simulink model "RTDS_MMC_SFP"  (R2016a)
settings: Solver=FixedStepAuto  StartTime=0.0  StopTime=0.4  RelTol=1e-3
PreLoadFcn:
  | % --- DO NOT REMOVE THIS CODE (2024.3.b1) ---
  |     % create Simulink variants
  |     if not(exist('variant_simulation', 'var'))
  |         variant_simulation = Simulink.Variant('SIMULINK_MODE==0');
  |     end
  |     if not(exist('variant_generation', 'var'))
  |         variant_generation = Simulink.Variant('SIMULINK_MODE==1');
  |     end
  | 
  |     % check SDK version
  |     required_lib_version = 3900.3;
  |     required_lib_ver_str = '2024.3';
  |     lib_path = [getenv('IX_SIMULINK_ACG_BB_3') '\simulink\blocks\BoomBox.slx'];
  |     if exist(lib_path, 'file')
  |         lib_version = str2double(Simulink.MDLInfo(lib_path).ModelVersion); % fullpath to avoid getting shadowing files
  |         if lib_version < required_lib_version || isnan(lib_version)
  |             error(['The model ''' bdroot ''' has been saved with a more recent version of ACG SDK (' required_lib_ver_str ') and might not work as expected. <a href="matlab:private_end_string = ''--- PLACE YOUR CODE BELOW THIS LINE ---'';private_fcn = get_param(bdroot, ''PreLoadFcn'');private_end_index = strfind(private_fcn, private_end_string);set_param(bdroot, ''PreLoadFcn'', strtrim(private_fcn(private_end_index(end)+length(private_end_string):end)));private_fcn = get_param(bdroot, ''PostLoadFcn'');private_end_index = strfind(private_fcn, private_end_string);set_param(bdroot, ''PostLoadFcn'', strtrim(private_fcn(private_end_index(end)+length(private_end_string):end)));private_fcn = get_param(bdroot, ''InitFcn'');private_end_index = strfind(private_fcn, private_end_string);set_param(bdroot, ''InitFcn'', strtrim(private_fcn(private_end_index(end)+length(private_end_string):end)));clear private_end_string private_fcn private_end_index;open(bdroot);">Click here</a> to continue anyway, or download the latest version of the SDK at <a href="www.imperix.com/downloads">www.imperix.ch/downloads</a>.']);
  |         end
  |     elseif exist(getenv('IX_SIMULINK_ACG_BB_3'), 'dir')
  |         error(['Library file for imperix ACG SDK not found in path ''' lib_path '''. Please try to re-install ACG SDK (<a href="www.imperix.com/downloads">www.imperix.ch/downloads</a>).']);
  |     else
  |         error('ACG SDK is not installed on this computer and the model will not work as expected. Please download ACG SDK at <a href="www.imperix.com/downloads">www.imperix.ch/downloads</a>, install it, and reopen the model.');
  |     end
  |     clear required_lib_version required_lib_ver_str lib_path lib_version;
  | 
  |     ix_acg_path = getenv('IX_SIMULINK_ACG_BB_3');
  |     addpath(fullfile(ix_acg_path, 'simulink\target'));
  |     addpath(fullfile(ix_acg_path, 'simulink\blocks'));
  |     addpath(fullfile(ix_acg_path, 'simulink\functions'));
  |     sl_refresh_customizations;
  |     clear ix_acg_path;
  | 
  |     % The SIMULINK_MODE variable is created in the base
  |     % workspace in the PostLoadFcn from the block whose id is kb0101
  |     % All opened models share a common variant configuration.
  | 
  |     Model_PreLoadFcn(bdroot);
  | % --- PLACE YOUR CODE BELOW THIS LINE ---
PostLoadFcn:
  | % --- DO NOT REMOVE THIS CODE (2024.3.b1) ---
  |     % change the execution mode of simulink depending on the radio button:
  |     if(strcmp('Automated Code Generation',get_param(Find_imperix_blocks(bdroot,'Configuration'),'SLMODE')))
  |         assignin('base', 'SIMULINK_MODE', 1);
  |     else
  |         assignin('base', 'SIMULINK_MODE', 0);
  |     end
  | 
  |     Model_PostLoadFcn(bdroot);
  | % --- PLACE YOUR CODE BELOW THIS LINE ---
InitFcn:
  | % --- DO NOT REMOVE THIS CODE (2024.3.b1) ---
  |     % check SDK version
  |     required_lib_version = 3900.3;
  |     required_lib_ver_str = '2024.3';
  |     lib_path = [getenv('IX_SIMULINK_ACG_BB_3') '\simulink\blocks\BoomBox.slx'];
  |     if exist(lib_path, 'file')
  |         lib_version = str2double(Simulink.MDLInfo(lib_path).ModelVersion); % fullpath to avoid getting shadowing files
  |         if lib_version < required_lib_version || isnan(lib_version)
  |             error(['The model ''' bdroot ''' has been saved with a more recent version of ACG SDK (' required_lib_ver_str ') and might not work as expected. <a href="matlab:private_end_string = ''--- PLACE YOUR CODE BELOW THIS LINE ---'';private_fcn = get_param(bdroot, ''PreLoadFcn'');private_end_index = strfind(private_fcn, private_end_string);set_param(bdroot, ''PreLoadFcn'', strtrim(private_fcn(private_end_index(end)+length(private_end_string):end)));private_fcn = get_param(bdroot, ''PostLoadFcn'');private_end_index = strfind(private_fcn, private_end_string);set_param(bdroot, ''PostLoadFcn'', strtrim(private_fcn(private_end_index(end)+length(private_end_string):end)));private_fcn = get_param(bdroot, ''InitFcn'');private_end_index = strfind(private_fcn, private_end_string);set_param(bdroot, ''InitFcn'', strtrim(private_fcn(private_end_index(end)+length(private_end_string):end)));clear private_end_string private_fcn private_end_index;open(bdroot);">Click here</a> to continue anyway, or download the latest version of the SDK at <a href="www.imperix.com/downloads">www.imperix.ch/downloads</a>.']);
  |         end
  |     elseif exist(getenv('IX_SIMULINK_ACG_BB_3'), 'dir')
  |         error(['Library file for imperix ACG SDK not found in path ''' lib_path '''. Please try to re-install ACG SDK (<a href="www.imperix.com/downloads">www.imperix.ch/downloads</a>).']);
  |     else
  |         error('ACG SDK is not installed on this computer and the model will not work as expected. Please download ACG SDK at <a href="www.imperix.com/downloads">www.imperix.ch/downloads</a>, install it, and reopen the model.');
  |     end
  |     clear required_lib_version required_lib_ver_str lib_path lib_version;
  | 
  |     Model_InitFcn(bdroot);
  | % --- PLACE YOUR CODE BELOW THIS LINE ---
model workspace (MAT data in the model file):
  CTRLPERIOD = 0.0002
  TSAMPLE = 2e-06
  global_CLK_number = 0
  global_INT_number = 1
  global_SVM_instance_id = 0
  global_can_baud_rate = '1000000'
  global_comp_time = 0.2
  global_cycle_delay = 8e-05
  global_ip_addresses : cell (value not decoded)
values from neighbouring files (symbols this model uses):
  Ki_Vleg = 1/Ti    (= 2.95256991686)    [RTDS_MMC_SFP_init.m]
  Kp_Vleg = Tn/Ti    (= 0.14880952381)    [RTDS_MMC_SFP_init.m]
  N = 4    [RTDS_MMC_SFP_init.m]
  scale_factor = 0.5^16    (= 1.52587890625e-05)    [RTDS_MMC_SFP_init.m]
  Tsw = 1/fsw    (= 0.0008)    [RTDS_MMC_SFP_init.m]
  Vsm_max = 250    [RTDS_MMC_SFP_init.m]
undefined symbols (not defined in the file or in its folder): B, Board, Box, channel, DT, lane, Micro, ns, PRO, RCP, TPI, Vf
libraries: BoomBox x183, simulink x55
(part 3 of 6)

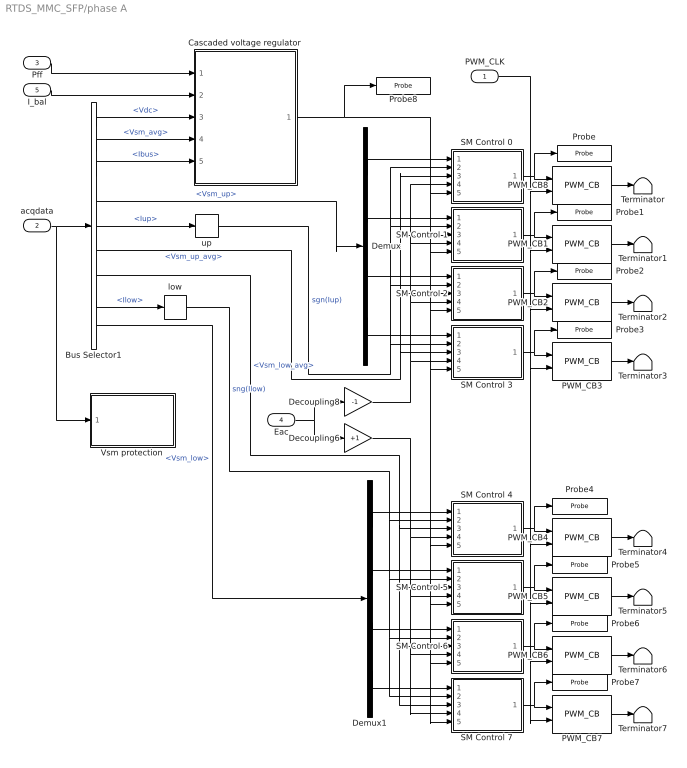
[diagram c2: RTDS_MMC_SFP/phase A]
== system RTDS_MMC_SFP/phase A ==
  PWM_CLK : Inport
  acqdata : Inport  Port=2
  Pff : Inport  Port=3
  Eac : Inport  Port=4
  I_bal : Inport  Port=5
  Bus Selector1 : BusSelector  OutputSignals=Vdc,A.Vsm.Vsm_avg,A.Ibus,A.Vsm.Vsm_up,A.Iup,A.Vsm.Vsm_up_avg,A.Vsm.Vsm_low_avg,A.Ilow,A.Vsm.Vsm_low
  Cascaded voltage regulator : Subsystem
  Decoupling6 : Gain  Gain=+1
  Decoupling8 : Gain  Gain=-1
  Demux : Demux
  Demux1 : Demux
  PWM_CB1 : BoomBox/PWM_CB  NB_BBX=0  OUTCONF=Single  PWM_OUT_SINGLE=lane 1 (channel 0L)  PWM_OUT_DUAL=channel 0 (lanes 0 & 1)  CARRIER=TRIANGLE  DUTY=0  DUTY_is_RT=on  PHASE=0.25  PHASE_is_RT=off  ENABLE_is_RT=off  RATE=Double-rate  ENABLE_DOUT=PWM signals  DEADTIME=400e-9  DEADTIME_SIM=off  LNorCH_NBR=1  CH_NBR=0  LN_NBR=1  Parameter16=0  KBID=kb0401
  PWM_CB2 : BoomBox/PWM_CB  NB_BBX=0  OUTCONF=Single  PWM_OUT_SINGLE=lane 2 (channel 1H)  PWM_OUT_DUAL=channel 0 (lanes 0 & 1)  CARRIER=TRIANGLE  DUTY=0  DUTY_is_RT=on  PHASE=0.5  PHASE_is_RT=off  ENABLE_is_RT=off  RATE=Double-rate  ENABLE_DOUT=PWM signals  DEADTIME=400e-9  DEADTIME_SIM=off  LNorCH_NBR=2  CH_NBR=0  LN_NBR=2  Parameter16=0  KBID=kb0401
  PWM_CB3 : BoomBox/PWM_CB  NB_BBX=0  OUTCONF=Single  PWM_OUT_SINGLE=lane 3 (channel 1L)  PWM_OUT_DUAL=channel 0 (lanes 0 & 1)  CARRIER=TRIANGLE  DUTY=0  DUTY_is_RT=on  PHASE=0.75  PHASE_is_RT=off  ENABLE_is_RT=off  RATE=Double-rate  ENABLE_DOUT=PWM signals  DEADTIME=400e-9  DEADTIME_SIM=off  LNorCH_NBR=3  CH_NBR=0  LN_NBR=3  Parameter16=0  KBID=kb0401
  PWM_CB4 : BoomBox/PWM_CB  NB_BBX=0  OUTCONF=Single  PWM_OUT_SINGLE=lane 4 (channel 2H)  PWM_OUT_DUAL=channel 0 (lanes 0 & 1)  CARRIER=TRIANGLE  DUTY=0  DUTY_is_RT=on  PHASE=0  PHASE_is_RT=off  ENABLE_is_RT=off  RATE=Double-rate  ENABLE_DOUT=PWM signals  DEADTIME=400e-9  DEADTIME_SIM=off  LNorCH_NBR=4  CH_NBR=0  LN_NBR=4  Parameter16=0  KBID=kb0401
  PWM_CB5 : BoomBox/PWM_CB  NB_BBX=0  OUTCONF=Single  PWM_OUT_SINGLE=lane 5 (channel 2L)  PWM_OUT_DUAL=channel 0 (lanes 0 & 1)  CARRIER=TRIANGLE  DUTY=0  DUTY_is_RT=on  PHASE=0.25  PHASE_is_RT=off  ENABLE_is_RT=off  RATE=Double-rate  ENABLE_DOUT=PWM signals  DEADTIME=400e-9  DEADTIME_SIM=off  LNorCH_NBR=5  CH_NBR=0  LN_NBR=5  Parameter16=0  KBID=kb0401
  PWM_CB6 : BoomBox/PWM_CB  NB_BBX=0  OUTCONF=Single  PWM_OUT_SINGLE=lane 6 (channel 3H)  PWM_OUT_DUAL=channel 0 (lanes 0 & 1)  CARRIER=TRIANGLE  DUTY=0  DUTY_is_RT=on  PHASE=0.5  PHASE_is_RT=off  ENABLE_is_RT=off  RATE=Double-rate  ENABLE_DOUT=PWM signals  DEADTIME=400e-9  DEADTIME_SIM=off  LNorCH_NBR=6  CH_NBR=0  LN_NBR=6  Parameter16=0  KBID=kb0401
  PWM_CB7 : BoomBox/PWM_CB  NB_BBX=0  OUTCONF=Single  PWM_OUT_SINGLE=lane 7 (channel 3L)  PWM_OUT_DUAL=channel 0 (lanes 0 & 1)  CARRIER=TRIANGLE  DUTY=0  DUTY_is_RT=on  PHASE=0.75  PHASE_is_RT=off  ENABLE_is_RT=off  RATE=Double-rate  ENABLE_DOUT=PWM signals  DEADTIME=400e-9  DEADTIME_SIM=off  LNorCH_NBR=7  CH_NBR=0  LN_NBR=7  Parameter16=0  KBID=kb0401
  PWM_CB8 : BoomBox/PWM_CB  NB_BBX=0  OUTCONF=Single  PWM_OUT_SINGLE=lane 0 (channel 0H)  PWM_OUT_DUAL=channel 0 (lanes 0 & 1)  CARRIER=TRIANGLE  DUTY=0  DUTY_is_RT=on  PHASE=0  PHASE_is_RT=off  ENABLE_is_RT=off  RATE=Double-rate  ENABLE_DOUT=PWM signals  DEADTIME=400e-9  DEADTIME_SIM=off  LNorCH_NBR=0  CH_NBR=0  LN_NBR=0  Parameter16=0  KBID=kb0401
  Probe : BoomBox/Probe  VARNAME=m_A0  EVALUATE=Literal  DATATYPE=single  CAN_ENABLED=off  CAN_ADDRESS=0  CAN_TX_FREQ=10  init_baudrate=0  CAN_BAUDRATE=1000000  can_endianness=Little-endian  ETH_ENABLED=off  ETH_PORT=2000  ETH_IP_LIST=IP address 0  eth_endianness=Little-endian  ETH_TX_FREQ=10  init_ip=0  KBID=kb0502  CAN_BIG_ENDIAN=0  ETH_BIG_ENDIAN=0  ETH_IP_SFCN=empty  CAN_MB_ID=0  ETH_MB_ID=1  RESIZE=0
  Probe1 : BoomBox/Probe  VARNAME=m_A1  EVALUATE=Literal  DATATYPE=single  CAN_ENABLED=off  CAN_ADDRESS=0  CAN_TX_FREQ=10  init_baudrate=0  CAN_BAUDRATE=1000000  can_endianness=Little-endian  ETH_ENABLED=off  ETH_PORT=2000  ETH_IP_LIST=IP address 0  eth_endianness=Little-endian  ETH_TX_FREQ=10  init_ip=0  KBID=kb0502  CAN_BIG_ENDIAN=0  ETH_BIG_ENDIAN=0  ETH_IP_SFCN=empty  CAN_MB_ID=0  ETH_MB_ID=1  RESIZE=0
  Probe2 : BoomBox/Probe  VARNAME=m_A2  EVALUATE=Literal  DATATYPE=single  CAN_ENABLED=off  CAN_ADDRESS=0  CAN_TX_FREQ=10  init_baudrate=0  CAN_BAUDRATE=1000000  can_endianness=Little-endian  ETH_ENABLED=off  ETH_PORT=2000  ETH_IP_LIST=IP address 0  eth_endianness=Little-endian  ETH_TX_FREQ=10  init_ip=0  KBID=kb0502  CAN_BIG_ENDIAN=0  ETH_BIG_ENDIAN=0  ETH_IP_SFCN=empty  CAN_MB_ID=0  ETH_MB_ID=1  RESIZE=0
  Probe3 : BoomBox/Probe  VARNAME=m_A3  EVALUATE=Literal  DATATYPE=single  CAN_ENABLED=off  CAN_ADDRESS=0  CAN_TX_FREQ=10  init_baudrate=0  CAN_BAUDRATE=1000000  can_endianness=Little-endian  ETH_ENABLED=off  ETH_PORT=2000  ETH_IP_LIST=IP address 0  eth_endianness=Little-endian  ETH_TX_FREQ=10  init_ip=0  KBID=kb0502  CAN_BIG_ENDIAN=0  ETH_BIG_ENDIAN=0  ETH_IP_SFCN=empty  CAN_MB_ID=0  ETH_MB_ID=1  RESIZE=0
  Probe4 : BoomBox/Probe  VARNAME=m_A4  EVALUATE=Literal  DATATYPE=single  CAN_ENABLED=off  CAN_ADDRESS=0  CAN_TX_FREQ=10  init_baudrate=0  CAN_BAUDRATE=1000000  can_endianness=Little-endian  ETH_ENABLED=off  ETH_PORT=2000  ETH_IP_LIST=IP address 0  eth_endianness=Little-endian  ETH_TX_FREQ=10  init_ip=0  KBID=kb0502  CAN_BIG_ENDIAN=0  ETH_BIG_ENDIAN=0  ETH_IP_SFCN=empty  CAN_MB_ID=0  ETH_MB_ID=1  RESIZE=0
  Probe5 : BoomBox/Probe  VARNAME=m_A5  EVALUATE=Literal  DATATYPE=single  CAN_ENABLED=off  CAN_ADDRESS=0  CAN_TX_FREQ=10  init_baudrate=0  CAN_BAUDRATE=1000000  can_endianness=Little-endian  ETH_ENABLED=off  ETH_PORT=2000  ETH_IP_LIST=IP address 0  eth_endianness=Little-endian  ETH_TX_FREQ=10  init_ip=0  KBID=kb0502  CAN_BIG_ENDIAN=0  ETH_BIG_ENDIAN=0  ETH_IP_SFCN=empty  CAN_MB_ID=0  ETH_MB_ID=1  RESIZE=0
  Probe6 : BoomBox/Probe  VARNAME=m_A6  EVALUATE=Literal  DATATYPE=single  CAN_ENABLED=off  CAN_ADDRESS=0  CAN_TX_FREQ=10  init_baudrate=0  CAN_BAUDRATE=1000000  can_endianness=Little-endian  ETH_ENABLED=off  ETH_PORT=2000  ETH_IP_LIST=IP address 0  eth_endianness=Little-endian  ETH_TX_FREQ=10  init_ip=0  KBID=kb0502  CAN_BIG_ENDIAN=0  ETH_BIG_ENDIAN=0  ETH_IP_SFCN=empty  CAN_MB_ID=0  ETH_MB_ID=1  RESIZE=0
  Probe7 : BoomBox/Probe  VARNAME=m_A7  EVALUATE=Literal  DATATYPE=single  CAN_ENABLED=off  CAN_ADDRESS=0  CAN_TX_FREQ=10  init_baudrate=0  CAN_BAUDRATE=1000000  can_endianness=Little-endian  ETH_ENABLED=off  ETH_PORT=2000  ETH_IP_LIST=IP address 0  eth_endianness=Little-endian  ETH_TX_FREQ=10  init_ip=0  KBID=kb0502  CAN_BIG_ENDIAN=0  ETH_BIG_ENDIAN=0  ETH_IP_SFCN=empty  CAN_MB_ID=0  ETH_MB_ID=1  RESIZE=0
  Probe8 : BoomBox/Probe  VARNAME=Edc_A  EVALUATE=Literal  DATATYPE=single  CAN_ENABLED=off  CAN_ADDRESS=0  CAN_TX_FREQ=10  init_baudrate=0  CAN_BAUDRATE=1000000  can_endianness=Little-endian  ETH_ENABLED=off  ETH_PORT=2000  ETH_IP_LIST=IP address 0  eth_endianness=Little-endian  ETH_TX_FREQ=10  init_ip=0  KBID=kb0502  CAN_BIG_ENDIAN=0  ETH_BIG_ENDIAN=0  ETH_IP_SFCN=empty  CAN_MB_ID=0  ETH_MB_ID=1  RESIZE=0
  SM Control 0 : Subsystem
  SM Control 1 : Subsystem
  SM Control 2 : Subsystem
  SM Control 3 : Subsystem
  SM Control 4 : Subsystem
  SM Control 5 : Subsystem
  SM Control 6 : Subsystem
  SM Control 7 : Subsystem
  Terminator{,1..7} (8 alike) : Terminator
  Vsm protection : Subsystem
  low : Signum
  up : Signum
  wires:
  low/1 -> SM Control 4/2(sign), SM Control 5/2(sign), SM Control 7/2(sign), SM Control 6/2(sign)  "sng(Ilow)"
  Bus Selector1/6 -> SM Control 3/3(Vsm_avg), SM Control 2/3(Vsm_avg), SM Control 1/3(Vsm_avg), SM Control 0/3(Vsm_avg)  "<Vsm_up_avg>"
  Demux1/1 -> SM Control 4/1(Vsm)
  Demux/3 -> SM Control 2/1(Vsm)
  Demux/2 -> SM Control 1/1(Vsm)
  Demux/4 -> SM Control 3/1(Vsm)
  Decoupling8/1 -> SM Control 3/4(Eac), SM Control 2/4(Eac), SM Control 1/4(Eac), SM Control 0/4(Eac)
  up/1 -> SM Control 3/2(sign), SM Control 2/2(sign), SM Control 1/2(sign), SM Control 0/2(sign)  "sgn(Iup)"
  acqdata/1 -> Vsm protection/1(acqdata), Bus Selector1/1
  Demux1/2 -> SM Control 5/1(Vsm)
  PWM_CLK/1 -> PWM_CB8/2, PWM_CB1/2, PWM_CB2/2, PWM_CB3/2, PWM_CB4/2, PWM_CB5/2, PWM_CB7/2, PWM_CB6/2
  SM Control 1/1(m) -> PWM_CB1/1, Probe1/1
  Demux1/4 -> SM Control 7/1(Vsm)
  SM Control 6/1(m) -> PWM_CB6/1, Probe6/1
  Decoupling6/1 -> SM Control 4/4(Eac), SM Control 5/4(Eac), SM Control 7/4(Eac), SM Control 6/4(Eac)
  Bus Selector1/7 -> SM Control 4/3(Vsm_avg), SM Control 5/3(Vsm_avg), SM Control 7/3(Vsm_avg), SM Control 6/3(Vsm_avg)  "<Vsm_low_avg>"
  Bus Selector1/8 -> low/1  "<Ilow>"
  Bus Selector1/9 -> Demux1/1  "<Vsm_low>"
  Demux/1 -> SM Control 0/1(Vsm)
  SM Control 5/1(m) -> PWM_CB5/1, Probe5/1
  SM Control 7/1(m) -> PWM_CB7/1, Probe7/1
  SM Control 3/1(m) -> PWM_CB3/1, Probe3/1
  Demux1/3 -> SM Control 6/1(Vsm)
  SM Control 0/1(m) -> Probe/1, PWM_CB8/1
  SM Control 2/1(m) -> PWM_CB2/1, Probe2/1
  SM Control 4/1(m) -> PWM_CB4/1, Probe4/1
  Bus Selector1/4 -> Demux/1  "<Vsm_up>"
  Bus Selector1/5 -> up/1  "<Iup>"
  Eac/1 -> Decoupling6/1, Decoupling8/1
  Cascaded voltage regulator/1(Edc) -> Probe8/1, SM Control 1/5(Edc), SM Control 2/5(Edc), SM Control 3/5(Edc), SM Control 4/5(Edc), SM Control 5/5(Edc), SM Control 7/5(Edc), SM Control 6/5(Edc), SM Control 0/5(Edc)
  Pff/1 -> Cascaded voltage regulator/1(Pff)
  I_bal/1 -> Cascaded voltage regulator/2(I_bal)
  Bus Selector1/1 -> Cascaded voltage regulator/3(Vdc)  "<Vdc>"
  Bus Selector1/2 -> Cascaded voltage regulator/4(Vsm_avg)  "<Vsm_avg>"
  Bus Selector1/3 -> Cascaded voltage regulator/5(Ibus)  "<Ibus>"
  PWM_CB8/1 -> Terminator/1
  PWM_CB1/1 -> Terminator1/1
  PWM_CB3/1 -> Terminator3/1
  PWM_CB2/1 -> Terminator2/1
  PWM_CB5/1 -> Terminator5/1
  PWM_CB4/1 -> Terminator4/1
  PWM_CB6/1 -> Terminator6/1
  PWM_CB7/1 -> Terminator7/1

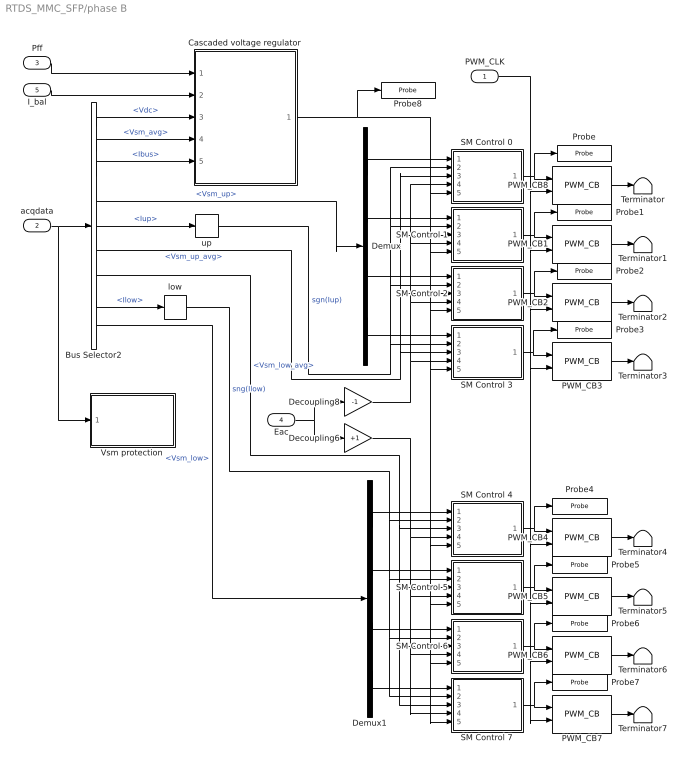
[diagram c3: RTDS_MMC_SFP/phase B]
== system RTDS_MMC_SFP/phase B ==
  PWM_CLK : Inport
  acqdata : Inport  Port=2
  Pff : Inport  Port=3
  Eac : Inport  Port=4
  I_bal : Inport  Port=5
  Bus Selector2 : BusSelector  OutputSignals=Vdc,B.Vsm.Vsm_avg,B.Ibus,B.Vsm.Vsm_up,B.Iup,B.Vsm.Vsm_up_avg,B.Vsm.Vsm_low_avg,B.Ilow,B.Vsm.Vsm_low
  Cascaded voltage regulator : Subsystem
  Decoupling6 : Gain  Gain=+1
  Decoupling8 : Gain  Gain=-1
  Demux : Demux
  Demux1 : Demux
  PWM_CB1 : BoomBox/PWM_CB  NB_BBX=0  OUTCONF=Single  PWM_OUT_SINGLE=lane 9 (channel 4L)  PWM_OUT_DUAL=channel 0 (lanes 0 & 1)  CARRIER=TRIANGLE  DUTY=0  DUTY_is_RT=on  PHASE=0.25  PHASE_is_RT=off  ENABLE_is_RT=off  RATE=Double-rate  ENABLE_DOUT=PWM signals  DEADTIME=400e-9  DEADTIME_SIM=off  LNorCH_NBR=9  CH_NBR=0  LN_NBR=9  Parameter16=0  KBID=kb0401
  PWM_CB2 : BoomBox/PWM_CB  NB_BBX=0  OUTCONF=Single  PWM_OUT_SINGLE=lane 10 (channel 5H)  PWM_OUT_DUAL=channel 0 (lanes 0 & 1)  CARRIER=TRIANGLE  DUTY=0  DUTY_is_RT=on  PHASE=0.5  PHASE_is_RT=off  ENABLE_is_RT=off  RATE=Double-rate  ENABLE_DOUT=PWM signals  DEADTIME=400e-9  DEADTIME_SIM=off  LNorCH_NBR=10  CH_NBR=0  LN_NBR=10  Parameter16=0  KBID=kb0401
  PWM_CB3 : BoomBox/PWM_CB  NB_BBX=0  OUTCONF=Single  PWM_OUT_SINGLE=lane 11 (channel 5L)  PWM_OUT_DUAL=channel 0 (lanes 0 & 1)  CARRIER=TRIANGLE  DUTY=0  DUTY_is_RT=on  PHASE=0.75  PHASE_is_RT=off  ENABLE_is_RT=off  RATE=Double-rate  ENABLE_DOUT=PWM signals  DEADTIME=400e-9  DEADTIME_SIM=off  LNorCH_NBR=11  CH_NBR=0  LN_NBR=11  Parameter16=0  KBID=kb0401
  PWM_CB4 : BoomBox/PWM_CB  NB_BBX=0  OUTCONF=Single  PWM_OUT_SINGLE=lane 12 (channel 6H)  PWM_OUT_DUAL=channel 0 (lanes 0 & 1)  CARRIER=TRIANGLE  DUTY=0  DUTY_is_RT=on  PHASE=0  PHASE_is_RT=off  ENABLE_is_RT=off  RATE=Double-rate  ENABLE_DOUT=PWM signals  DEADTIME=400e-9  DEADTIME_SIM=off  LNorCH_NBR=12  CH_NBR=0  LN_NBR=12  Parameter16=0  KBID=kb0401
  PWM_CB5 : BoomBox/PWM_CB  NB_BBX=0  OUTCONF=Single  PWM_OUT_SINGLE=lane 13 (channel 6L)  PWM_OUT_DUAL=channel 0 (lanes 0 & 1)  CARRIER=TRIANGLE  DUTY=0  DUTY_is_RT=on  PHASE=0.25  PHASE_is_RT=off  ENABLE_is_RT=off  RATE=Double-rate  ENABLE_DOUT=PWM signals  DEADTIME=400e-9  DEADTIME_SIM=off  LNorCH_NBR=13  CH_NBR=0  LN_NBR=13  Parameter16=0  KBID=kb0401
  PWM_CB6 : BoomBox/PWM_CB  NB_BBX=0  OUTCONF=Single  PWM_OUT_SINGLE=lane 14 (channel 7H)  PWM_OUT_DUAL=channel 0 (lanes 0 & 1)  CARRIER=TRIANGLE  DUTY=0  DUTY_is_RT=on  PHASE=0.5  PHASE_is_RT=off  ENABLE_is_RT=off  RATE=Double-rate  ENABLE_DOUT=PWM signals  DEADTIME=400e-9  DEADTIME_SIM=off  LNorCH_NBR=14  CH_NBR=0  LN_NBR=14  Parameter16=0  KBID=kb0401
  PWM_CB7 : BoomBox/PWM_CB  NB_BBX=0  OUTCONF=Single  PWM_OUT_SINGLE=lane 15 (channel 7L)  PWM_OUT_DUAL=channel 0 (lanes 0 & 1)  CARRIER=TRIANGLE  DUTY=0  DUTY_is_RT=on  PHASE=0.75  PHASE_is_RT=off  ENABLE_is_RT=off  RATE=Double-rate  ENABLE_DOUT=PWM signals  DEADTIME=400e-9  DEADTIME_SIM=off  LNorCH_NBR=15  CH_NBR=0  LN_NBR=15  Parameter16=0  KBID=kb0401
  PWM_CB8 : BoomBox/PWM_CB  NB_BBX=0  OUTCONF=Single  PWM_OUT_SINGLE=lane 8 (channel 4H)  PWM_OUT_DUAL=channel 0 (lanes 0 & 1)  CARRIER=TRIANGLE  DUTY=0  DUTY_is_RT=on  PHASE=0  PHASE_is_RT=off  ENABLE_is_RT=off  RATE=Double-rate  ENABLE_DOUT=PWM signals  DEADTIME=400e-9  DEADTIME_SIM=off  LNorCH_NBR=8  CH_NBR=0  LN_NBR=8  Parameter16=0  KBID=kb0401
  Probe : BoomBox/Probe  VARNAME=m_B0  EVALUATE=Literal  DATATYPE=single  CAN_ENABLED=off  CAN_ADDRESS=0  CAN_TX_FREQ=10  init_baudrate=0  CAN_BAUDRATE=1000000  can_endianness=Little-endian  ETH_ENABLED=off  ETH_PORT=2000  ETH_IP_LIST=IP address 0  eth_endianness=Little-endian  ETH_TX_FREQ=10  init_ip=0  KBID=kb0502  CAN_BIG_ENDIAN=0  ETH_BIG_ENDIAN=0  ETH_IP_SFCN=empty  CAN_MB_ID=0  ETH_MB_ID=1  RESIZE=0
  Probe1 : BoomBox/Probe  VARNAME=m_B1  EVALUATE=Literal  DATATYPE=single  CAN_ENABLED=off  CAN_ADDRESS=0  CAN_TX_FREQ=10  init_baudrate=0  CAN_BAUDRATE=1000000  can_endianness=Little-endian  ETH_ENABLED=off  ETH_PORT=2000  ETH_IP_LIST=IP address 0  eth_endianness=Little-endian  ETH_TX_FREQ=10  init_ip=0  KBID=kb0502  CAN_BIG_ENDIAN=0  ETH_BIG_ENDIAN=0  ETH_IP_SFCN=empty  CAN_MB_ID=0  ETH_MB_ID=1  RESIZE=0
  Probe2 : BoomBox/Probe  VARNAME=m_B2  EVALUATE=Literal  DATATYPE=single  CAN_ENABLED=off  CAN_ADDRESS=0  CAN_TX_FREQ=10  init_baudrate=0  CAN_BAUDRATE=1000000  can_endianness=Little-endian  ETH_ENABLED=off  ETH_PORT=2000  ETH_IP_LIST=IP address 0  eth_endianness=Little-endian  ETH_TX_FREQ=10  init_ip=0  KBID=kb0502  CAN_BIG_ENDIAN=0  ETH_BIG_ENDIAN=0  ETH_IP_SFCN=empty  CAN_MB_ID=0  ETH_MB_ID=1  RESIZE=0
  Probe3 : BoomBox/Probe  VARNAME=m_B3  EVALUATE=Literal  DATATYPE=single  CAN_ENABLED=off  CAN_ADDRESS=0  CAN_TX_FREQ=10  init_baudrate=0  CAN_BAUDRATE=1000000  can_endianness=Little-endian  ETH_ENABLED=off  ETH_PORT=2000  ETH_IP_LIST=IP address 0  eth_endianness=Little-endian  ETH_TX_FREQ=10  init_ip=0  KBID=kb0502  CAN_BIG_ENDIAN=0  ETH_BIG_ENDIAN=0  ETH_IP_SFCN=empty  CAN_MB_ID=0  ETH_MB_ID=1  RESIZE=0
  Probe4 : BoomBox/Probe  VARNAME=m_B4  EVALUATE=Literal  DATATYPE=single  CAN_ENABLED=off  CAN_ADDRESS=0  CAN_TX_FREQ=10  init_baudrate=0  CAN_BAUDRATE=1000000  can_endianness=Little-endian  ETH_ENABLED=off  ETH_PORT=2000  ETH_IP_LIST=IP address 0  eth_endianness=Little-endian  ETH_TX_FREQ=10  init_ip=0  KBID=kb0502  CAN_BIG_ENDIAN=0  ETH_BIG_ENDIAN=0  ETH_IP_SFCN=empty  CAN_MB_ID=0  ETH_MB_ID=1  RESIZE=0
  Probe5 : BoomBox/Probe  VARNAME=m_B5  EVALUATE=Literal  DATATYPE=single  CAN_ENABLED=off  CAN_ADDRESS=0  CAN_TX_FREQ=10  init_baudrate=0  CAN_BAUDRATE=1000000  can_endianness=Little-endian  ETH_ENABLED=off  ETH_PORT=2000  ETH_IP_LIST=IP address 0  eth_endianness=Little-endian  ETH_TX_FREQ=10  init_ip=0  KBID=kb0502  CAN_BIG_ENDIAN=0  ETH_BIG_ENDIAN=0  ETH_IP_SFCN=empty  CAN_MB_ID=0  ETH_MB_ID=1  RESIZE=0
  Probe6 : BoomBox/Probe  VARNAME=m_B6  EVALUATE=Literal  DATATYPE=single  CAN_ENABLED=off  CAN_ADDRESS=0  CAN_TX_FREQ=10  init_baudrate=0  CAN_BAUDRATE=1000000  can_endianness=Little-endian  ETH_ENABLED=off  ETH_PORT=2000  ETH_IP_LIST=IP address 0  eth_endianness=Little-endian  ETH_TX_FREQ=10  init_ip=0  KBID=kb0502  CAN_BIG_ENDIAN=0  ETH_BIG_ENDIAN=0  ETH_IP_SFCN=empty  CAN_MB_ID=0  ETH_MB_ID=1  RESIZE=0
  Probe7 : BoomBox/Probe  VARNAME=m_B7  EVALUATE=Literal  DATATYPE=single  CAN_ENABLED=off  CAN_ADDRESS=0  CAN_TX_FREQ=10  init_baudrate=0  CAN_BAUDRATE=1000000  can_endianness=Little-endian  ETH_ENABLED=off  ETH_PORT=2000  ETH_IP_LIST=IP address 0  eth_endianness=Little-endian  ETH_TX_FREQ=10  init_ip=0  KBID=kb0502  CAN_BIG_ENDIAN=0  ETH_BIG_ENDIAN=0  ETH_IP_SFCN=empty  CAN_MB_ID=0  ETH_MB_ID=1  RESIZE=0
  Probe8 : BoomBox/Probe  VARNAME=Edc_B  EVALUATE=Literal  DATATYPE=single  CAN_ENABLED=off  CAN_ADDRESS=0  CAN_TX_FREQ=10  init_baudrate=0  CAN_BAUDRATE=1000000  can_endianness=Little-endian  ETH_ENABLED=off  ETH_PORT=2000  ETH_IP_LIST=IP address 0  eth_endianness=Little-endian  ETH_TX_FREQ=10  init_ip=0  KBID=kb0502  CAN_BIG_ENDIAN=0  ETH_BIG_ENDIAN=0  ETH_IP_SFCN=empty  CAN_MB_ID=0  ETH_MB_ID=1  RESIZE=0
  SM Control 0 : Subsystem
  SM Control 1 : Subsystem
  SM Control 2 : Subsystem
  SM Control 3 : Subsystem
  SM Control 4 : Subsystem
  SM Control 5 : Subsystem
  SM Control 6 : Subsystem
  SM Control 7 : Subsystem
  Terminator{,1..7} (8 alike) : Terminator
  Vsm protection : Subsystem
  low : Signum
  up : Signum
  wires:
  Bus Selector2/3 -> Cascaded voltage regulator/5(Ibus)  "<Ibus>"
  Bus Selector2/2 -> Cascaded voltage regulator/4(Vsm_avg)  "<Vsm_avg>"
  Bus Selector2/1 -> Cascaded voltage regulator/3(Vdc)  "<Vdc>"
  I_bal/1 -> Cascaded voltage regulator/2(I_bal)
  Pff/1 -> Cascaded voltage regulator/1(Pff)
  Cascaded voltage regulator/1(Edc) -> Probe8/1, SM Control 0/5(Edc), SM Control 1/5(Edc), SM Control 2/5(Edc), SM Control 3/5(Edc), SM Control 4/5(Edc), SM Control 5/5(Edc), SM Control 7/5(Edc), SM Control 6/5(Edc)
  Eac/1 -> Decoupling8/1, Decoupling6/1
  Bus Selector2/5 -> up/1  "<Iup>"
  Bus Selector2/4 -> Demux/1  "<Vsm_up>"
  SM Control 4/1(m) -> PWM_CB4/1, Probe4/1
  SM Control 2/1(m) -> PWM_CB2/1, Probe2/1
  SM Control 0/1(m) -> PWM_CB8/1, Probe/1
  Demux1/3 -> SM Control 6/1(Vsm)
  SM Control 3/1(m) -> PWM_CB3/1, Probe3/1
  SM Control 7/1(m) -> PWM_CB7/1, Probe7/1
  SM Control 5/1(m) -> PWM_CB5/1, Probe5/1
  Demux/1 -> SM Control 0/1(Vsm)
  Bus Selector2/9 -> Demux1/1  "<Vsm_low>"
  Bus Selector2/8 -> low/1  "<Ilow>"
  Bus Selector2/7 -> SM Control 4/3(Vsm_avg), SM Control 5/3(Vsm_avg), SM Control 7/3(Vsm_avg), SM Control 6/3(Vsm_avg)  "<Vsm_low_avg>"
  Decoupling6/1 -> SM Control 4/4(Eac), SM Control 5/4(Eac), SM Control 7/4(Eac), SM Control 6/4(Eac)
  SM Control 6/1(m) -> PWM_CB6/1, Probe6/1
  Demux1/4 -> SM Control 7/1(Vsm)
  SM Control 1/1(m) -> PWM_CB1/1, Probe1/1
  PWM_CLK/1 -> PWM_CB8/2, PWM_CB1/2, PWM_CB2/2, PWM_CB3/2, PWM_CB4/2, PWM_CB5/2, PWM_CB6/2, PWM_CB7/2
  Demux1/2 -> SM Control 5/1(Vsm)
  acqdata/1 -> Vsm protection/1(acqdata), Bus Selector2/1
  up/1 -> SM Control 3/2(sign), SM Control 2/2(sign), SM Control 1/2(sign), SM Control 0/2(sign)  "sgn(Iup)"
  Decoupling8/1 -> SM Control 3/4(Eac), SM Control 2/4(Eac), SM Control 1/4(Eac), SM Control 0/4(Eac)
  Demux/4 -> SM Control 3/1(Vsm)
  Demux/2 -> SM Control 1/1(Vsm)
  Demux/3 -> SM Control 2/1(Vsm)
  Demux1/1 -> SM Control 4/1(Vsm)
  Bus Selector2/6 -> SM Control 3/3(Vsm_avg), SM Control 2/3(Vsm_avg), SM Control 1/3(Vsm_avg), SM Control 0/3(Vsm_avg)  "<Vsm_up_avg>"
  low/1 -> SM Control 4/2(sign), SM Control 5/2(sign), SM Control 7/2(sign), SM Control 6/2(sign)  "sng(Ilow)"
  PWM_CB8/1 -> Terminator/1
  PWM_CB1/1 -> Terminator1/1
  PWM_CB2/1 -> Terminator2/1
  PWM_CB3/1 -> Terminator3/1
  PWM_CB4/1 -> Terminator4/1
  PWM_CB5/1 -> Terminator5/1
  PWM_CB6/1 -> Terminator6/1
  PWM_CB7/1 -> Terminator7/1

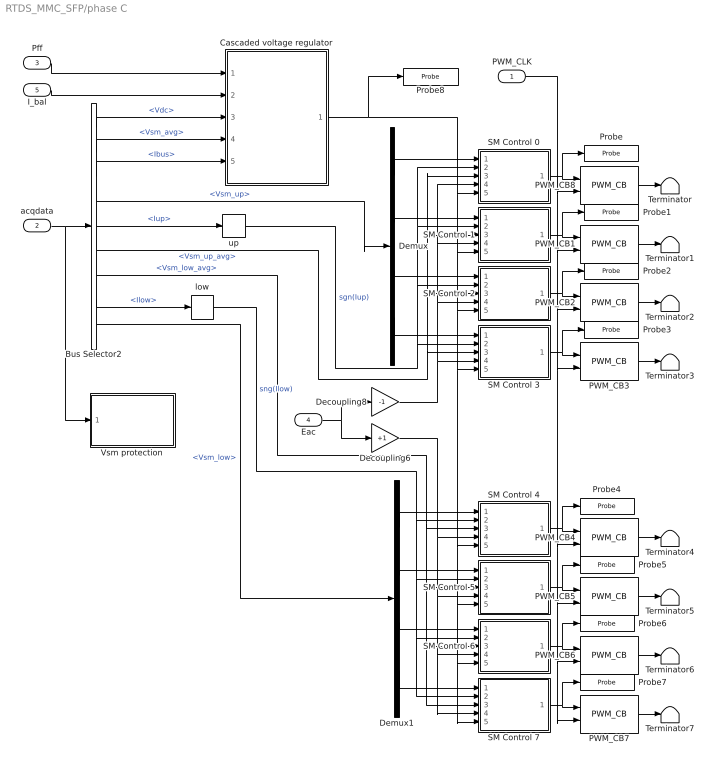
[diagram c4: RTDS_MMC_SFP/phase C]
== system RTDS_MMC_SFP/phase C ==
  PWM_CLK : Inport
  acqdata : Inport  Port=2
  Pff : Inport  Port=3
  Eac : Inport  Port=4
  I_bal : Inport  Port=5
  Bus Selector2 : BusSelector  OutputSignals=Vdc,C.Vsm.Vsm_avg,C.Ibus,C.Vsm.Vsm_up,C.Iup,C.Vsm.Vsm_up_avg,C.Vsm.Vsm_low_avg,C.Ilow,C.Vsm.Vsm_low
  Cascaded voltage regulator : Subsystem
  Decoupling6 : Gain  Gain=+1
  Decoupling8 : Gain  Gain=-1
  Demux : Demux
  Demux1 : Demux
  PWM_CB1 : BoomBox/PWM_CB  NB_BBX=0  OUTCONF=Single  PWM_OUT_SINGLE=lane 17 (channel 8L)  PWM_OUT_DUAL=channel 0 (lanes 0 & 1)  CARRIER=TRIANGLE  DUTY=0  DUTY_is_RT=on  PHASE=0.25  PHASE_is_RT=off  ENABLE_is_RT=off  RATE=Double-rate  ENABLE_DOUT=PWM signals  DEADTIME=400e-9  DEADTIME_SIM=off  LNorCH_NBR=17  CH_NBR=0  LN_NBR=17  Parameter16=0  KBID=kb0401
  PWM_CB2 : BoomBox/PWM_CB  NB_BBX=0  OUTCONF=Single  PWM_OUT_SINGLE=lane 18 (channel 9H)  PWM_OUT_DUAL=channel 0 (lanes 0 & 1)  CARRIER=TRIANGLE  DUTY=0  DUTY_is_RT=on  PHASE=0.5  PHASE_is_RT=off  ENABLE_is_RT=off  RATE=Double-rate  ENABLE_DOUT=PWM signals  DEADTIME=400e-9  DEADTIME_SIM=off  LNorCH_NBR=18  CH_NBR=0  LN_NBR=18  Parameter16=0  KBID=kb0401
  PWM_CB3 : BoomBox/PWM_CB  NB_BBX=0  OUTCONF=Single  PWM_OUT_SINGLE=lane 19 (channel 9L)  PWM_OUT_DUAL=channel 0 (lanes 0 & 1)  CARRIER=TRIANGLE  DUTY=0  DUTY_is_RT=on  PHASE=0.75  PHASE_is_RT=off  ENABLE_is_RT=off  RATE=Double-rate  ENABLE_DOUT=PWM signals  DEADTIME=400e-9  DEADTIME_SIM=off  LNorCH_NBR=19  CH_NBR=0  LN_NBR=19  Parameter16=0  KBID=kb0401
  PWM_CB4 : BoomBox/PWM_CB  NB_BBX=0  OUTCONF=Single  PWM_OUT_SINGLE=lane 20 (channel 10H)  PWM_OUT_DUAL=channel 0 (lanes 0 & 1)  CARRIER=TRIANGLE  DUTY=0  DUTY_is_RT=on  PHASE=0  PHASE_is_RT=off  ENABLE_is_RT=off  RATE=Double-rate  ENABLE_DOUT=PWM signals  DEADTIME=400e-9  DEADTIME_SIM=off  LNorCH_NBR=20  CH_NBR=0  LN_NBR=20  Parameter16=0  KBID=kb0401
  PWM_CB5 : BoomBox/PWM_CB  NB_BBX=0  OUTCONF=Single  PWM_OUT_SINGLE=lane 21 (channel 10L)  PWM_OUT_DUAL=channel 0 (lanes 0 & 1)  CARRIER=TRIANGLE  DUTY=0  DUTY_is_RT=on  PHASE=0.25  PHASE_is_RT=off  ENABLE_is_RT=off  RATE=Double-rate  ENABLE_DOUT=PWM signals  DEADTIME=400e-9  DEADTIME_SIM=off  LNorCH_NBR=21  CH_NBR=0  LN_NBR=21  Parameter16=0  KBID=kb0401
  PWM_CB6 : BoomBox/PWM_CB  NB_BBX=0  OUTCONF=Single  PWM_OUT_SINGLE=lane 22 (channel 11H)  PWM_OUT_DUAL=channel 0 (lanes 0 & 1)  CARRIER=TRIANGLE  DUTY=0  DUTY_is_RT=on  PHASE=0.5  PHASE_is_RT=off  ENABLE_is_RT=off  RATE=Double-rate  ENABLE_DOUT=PWM signals  DEADTIME=400e-9  DEADTIME_SIM=off  LNorCH_NBR=22  CH_NBR=0  LN_NBR=22  Parameter16=0  KBID=kb0401
  PWM_CB7 : BoomBox/PWM_CB  NB_BBX=0  OUTCONF=Single  PWM_OUT_SINGLE=lane 23 (channel 11L)  PWM_OUT_DUAL=channel 0 (lanes 0 & 1)  CARRIER=TRIANGLE  DUTY=0  DUTY_is_RT=on  PHASE=0.75  PHASE_is_RT=off  ENABLE_is_RT=off  RATE=Double-rate  ENABLE_DOUT=PWM signals  DEADTIME=400e-9  DEADTIME_SIM=off  LNorCH_NBR=23  CH_NBR=0  LN_NBR=23  Parameter16=0  KBID=kb0401
  PWM_CB8 : BoomBox/PWM_CB  NB_BBX=0  OUTCONF=Single  PWM_OUT_SINGLE=lane 16 (channel 8H)  PWM_OUT_DUAL=channel 0 (lanes 0 & 1)  CARRIER=TRIANGLE  DUTY=0  DUTY_is_RT=on  PHASE=0  PHASE_is_RT=off  ENABLE_is_RT=off  RATE=Double-rate  ENABLE_DOUT=PWM signals  DEADTIME=400e-9  DEADTIME_SIM=off  LNorCH_NBR=16  CH_NBR=0  LN_NBR=16  Parameter16=0  KBID=kb0401
  Probe : BoomBox/Probe  VARNAME=m_C0  EVALUATE=Literal  DATATYPE=single  CAN_ENABLED=off  CAN_ADDRESS=0  CAN_TX_FREQ=10  init_baudrate=0  CAN_BAUDRATE=1000000  can_endianness=Little-endian  ETH_ENABLED=off  ETH_PORT=2000  ETH_IP_LIST=IP address 0  eth_endianness=Little-endian  ETH_TX_FREQ=10  init_ip=0  KBID=kb0502  CAN_BIG_ENDIAN=0  ETH_BIG_ENDIAN=0  ETH_IP_SFCN=empty  CAN_MB_ID=0  ETH_MB_ID=1  RESIZE=0
  Probe1 : BoomBox/Probe  VARNAME=m_C1  EVALUATE=Literal  DATATYPE=single  CAN_ENABLED=off  CAN_ADDRESS=0  CAN_TX_FREQ=10  init_baudrate=0  CAN_BAUDRATE=1000000  can_endianness=Little-endian  ETH_ENABLED=off  ETH_PORT=2000  ETH_IP_LIST=IP address 0  eth_endianness=Little-endian  ETH_TX_FREQ=10  init_ip=0  KBID=kb0502  CAN_BIG_ENDIAN=0  ETH_BIG_ENDIAN=0  ETH_IP_SFCN=empty  CAN_MB_ID=0  ETH_MB_ID=1  RESIZE=0
  Probe2 : BoomBox/Probe  VARNAME=m_C2  EVALUATE=Literal  DATATYPE=single  CAN_ENABLED=off  CAN_ADDRESS=0  CAN_TX_FREQ=10  init_baudrate=0  CAN_BAUDRATE=1000000  can_endianness=Little-endian  ETH_ENABLED=off  ETH_PORT=2000  ETH_IP_LIST=IP address 0  eth_endianness=Little-endian  ETH_TX_FREQ=10  init_ip=0  KBID=kb0502  CAN_BIG_ENDIAN=0  ETH_BIG_ENDIAN=0  ETH_IP_SFCN=empty  CAN_MB_ID=0  ETH_MB_ID=1  RESIZE=0
  Probe3 : BoomBox/Probe  VARNAME=m_C3  EVALUATE=Literal  DATATYPE=single  CAN_ENABLED=off  CAN_ADDRESS=0  CAN_TX_FREQ=10  init_baudrate=0  CAN_BAUDRATE=1000000  can_endianness=Little-endian  ETH_ENABLED=off  ETH_PORT=2000  ETH_IP_LIST=IP address 0  eth_endianness=Little-endian  ETH_TX_FREQ=10  init_ip=0  KBID=kb0502  CAN_BIG_ENDIAN=0  ETH_BIG_ENDIAN=0  ETH_IP_SFCN=empty  CAN_MB_ID=0  ETH_MB_ID=1  RESIZE=0
  Probe4 : BoomBox/Probe  VARNAME=m_C4  EVALUATE=Literal  DATATYPE=single  CAN_ENABLED=off  CAN_ADDRESS=0  CAN_TX_FREQ=10  init_baudrate=0  CAN_BAUDRATE=1000000  can_endianness=Little-endian  ETH_ENABLED=off  ETH_PORT=2000  ETH_IP_LIST=IP address 0  eth_endianness=Little-endian  ETH_TX_FREQ=10  init_ip=0  KBID=kb0502  CAN_BIG_ENDIAN=0  ETH_BIG_ENDIAN=0  ETH_IP_SFCN=empty  CAN_MB_ID=0  ETH_MB_ID=1  RESIZE=0
  Probe5 : BoomBox/Probe  VARNAME=m_C5  EVALUATE=Literal  DATATYPE=single  CAN_ENABLED=off  CAN_ADDRESS=0  CAN_TX_FREQ=10  init_baudrate=0  CAN_BAUDRATE=1000000  can_endianness=Little-endian  ETH_ENABLED=off  ETH_PORT=2000  ETH_IP_LIST=IP address 0  eth_endianness=Little-endian  ETH_TX_FREQ=10  init_ip=0  KBID=kb0502  CAN_BIG_ENDIAN=0  ETH_BIG_ENDIAN=0  ETH_IP_SFCN=empty  CAN_MB_ID=0  ETH_MB_ID=1  RESIZE=0
  Probe6 : BoomBox/Probe  VARNAME=m_C6  EVALUATE=Literal  DATATYPE=single  CAN_ENABLED=off  CAN_ADDRESS=0  CAN_TX_FREQ=10  init_baudrate=0  CAN_BAUDRATE=1000000  can_endianness=Little-endian  ETH_ENABLED=off  ETH_PORT=2000  ETH_IP_LIST=IP address 0  eth_endianness=Little-endian  ETH_TX_FREQ=10  init_ip=0  KBID=kb0502  CAN_BIG_ENDIAN=0  ETH_BIG_ENDIAN=0  ETH_IP_SFCN=empty  CAN_MB_ID=0  ETH_MB_ID=1  RESIZE=0
  Probe7 : BoomBox/Probe  VARNAME=m_C7  EVALUATE=Literal  DATATYPE=single  CAN_ENABLED=off  CAN_ADDRESS=0  CAN_TX_FREQ=10  init_baudrate=0  CAN_BAUDRATE=1000000  can_endianness=Little-endian  ETH_ENABLED=off  ETH_PORT=2000  ETH_IP_LIST=IP address 0  eth_endianness=Little-endian  ETH_TX_FREQ=10  init_ip=0  KBID=kb0502  CAN_BIG_ENDIAN=0  ETH_BIG_ENDIAN=0  ETH_IP_SFCN=empty  CAN_MB_ID=0  ETH_MB_ID=1  RESIZE=0
  Probe8 : BoomBox/Probe  VARNAME=Edc_C  EVALUATE=Literal  DATATYPE=single  CAN_ENABLED=off  CAN_ADDRESS=0  CAN_TX_FREQ=10  init_baudrate=0  CAN_BAUDRATE=1000000  can_endianness=Little-endian  ETH_ENABLED=off  ETH_PORT=2000  ETH_IP_LIST=IP address 0  eth_endianness=Little-endian  ETH_TX_FREQ=10  init_ip=0  KBID=kb0502  CAN_BIG_ENDIAN=0  ETH_BIG_ENDIAN=0  ETH_IP_SFCN=empty  CAN_MB_ID=0  ETH_MB_ID=1  RESIZE=0
  SM Control 0 : Subsystem
  SM Control 1 : Subsystem
  SM Control 2 : Subsystem
  SM Control 3 : Subsystem
  SM Control 4 : Subsystem
  SM Control 5 : Subsystem
  SM Control 6 : Subsystem
  SM Control 7 : Subsystem
  Terminator{,1..7} (8 alike) : Terminator
  Vsm protection : Subsystem
  low : Signum
  up : Signum
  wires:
  low/1 -> SM Control 4/2(sign), SM Control 5/2(sign), SM Control 7/2(sign), SM Control 6/2(sign)  "sng(Ilow)"
  Bus Selector2/6 -> SM Control 3/3(Vsm_avg), SM Control 2/3(Vsm_avg), SM Control 1/3(Vsm_avg), SM Control 0/3(Vsm_avg)  "<Vsm_up_avg>"
  Demux1/1 -> SM Control 4/1(Vsm)
  Demux/3 -> SM Control 2/1(Vsm)
  Demux/2 -> SM Control 1/1(Vsm)
  Demux/4 -> SM Control 3/1(Vsm)
  Decoupling8/1 -> SM Control 3/4(Eac), SM Control 2/4(Eac), SM Control 1/4(Eac), SM Control 0/4(Eac)
  up/1 -> SM Control 3/2(sign), SM Control 2/2(sign), SM Control 0/2(sign), SM Control 1/2(sign)  "sgn(Iup)"
  acqdata/1 -> Vsm protection/1(acqdata), Bus Selector2/1
  Demux1/2 -> SM Control 5/1(Vsm)
  PWM_CLK/1 -> PWM_CB8/2, PWM_CB1/2, PWM_CB2/2, PWM_CB3/2, PWM_CB4/2, PWM_CB5/2, PWM_CB7/2, PWM_CB6/2
  SM Control 1/1(m) -> PWM_CB1/1, Probe1/1
  Demux1/4 -> SM Control 7/1(Vsm)
  SM Control 6/1(m) -> PWM_CB6/1, Probe6/1
  Decoupling6/1 -> SM Control 4/4(Eac), SM Control 5/4(Eac), SM Control 7/4(Eac), SM Control 6/4(Eac)
  Bus Selector2/7 -> SM Control 4/3(Vsm_avg), SM Control 5/3(Vsm_avg), SM Control 7/3(Vsm_avg), SM Control 6/3(Vsm_avg)  "<Vsm_low_avg>"
  Bus Selector2/8 -> low/1  "<Ilow>"
  Bus Selector2/9 -> Demux1/1  "<Vsm_low>"
  Demux/1 -> SM Control 0/1(Vsm)
  SM Control 5/1(m) -> PWM_CB5/1, Probe5/1
  SM Control 7/1(m) -> PWM_CB7/1, Probe7/1
  SM Control 3/1(m) -> PWM_CB3/1, Probe3/1
  Demux1/3 -> SM Control 6/1(Vsm)
  SM Control 0/1(m) -> PWM_CB8/1, Probe/1
  SM Control 2/1(m) -> PWM_CB2/1, Probe2/1
  SM Control 4/1(m) -> PWM_CB4/1, Probe4/1
  Bus Selector2/4 -> Demux/1  "<Vsm_up>"
  Bus Selector2/5 -> up/1  "<Iup>"
  Eac/1 -> Decoupling6/1, Decoupling8/1
  Pff/1 -> Cascaded voltage regulator/1(Pff)
  I_bal/1 -> Cascaded voltage regulator/2(I_bal)
  Bus Selector2/1 -> Cascaded voltage regulator/3(Vdc)  "<Vdc>"
  Bus Selector2/2 -> Cascaded voltage regulator/4(Vsm_avg)  "<Vsm_avg>"
  Bus Selector2/3 -> Cascaded voltage regulator/5(Ibus)  "<Ibus>"
  Cascaded voltage regulator/1(Edc) -> Probe8/1, SM Control 0/5(Edc), SM Control 1/5(Edc), SM Control 2/5(Edc), SM Control 3/5(Edc), SM Control 4/5(Edc), SM Control 5/5(Edc), SM Control 7/5(Edc), SM Control 6/5(Edc)
  PWM_CB8/1 -> Terminator/1
  PWM_CB1/1 -> Terminator1/1
  PWM_CB2/1 -> Terminator2/1
  PWM_CB3/1 -> Terminator3/1
  PWM_CB4/1 -> Terminator4/1
  PWM_CB5/1 -> Terminator5/1
  PWM_CB6/1 -> Terminator6/1
  PWM_CB7/1 -> Terminator7/1

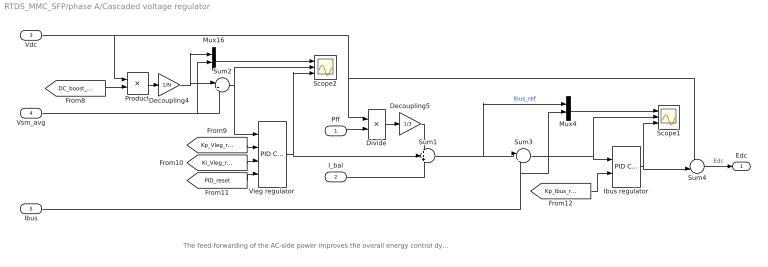
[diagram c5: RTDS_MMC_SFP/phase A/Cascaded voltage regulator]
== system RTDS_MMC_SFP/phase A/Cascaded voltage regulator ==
  note: The feed-forwarding of the AC-side power improves the overall energy control dynamics.
  Pff : Inport
  I_bal : Inport  Port=2
  Vdc : Inport  Port=3
  Vsm_avg : Inport  Port=4
  Ibus : Inport  Port=5
  Decoupling4 : Gain  Gain=1/N
  Decoupling5 : Gain  Gain=1/3
  Divide : Product  Inputs=/*
  Ibus regulator : simulink/Continuous/PID Controller  Controller=P  TimeDomain=Discrete-time  SampleTime=-1  IntegratorMethod=Forward Euler  FilterMethod=Forward Euler  Form=Parallel  UseFilter=on  ControllerParametersSource=external  P=8  I=0.5  D=0  N=100  InitialConditionSource=internal  InitialConditionForIntegrator=0  InitialConditionForFilter=0  ExternalReset=none  LimitOutput=off  UpperSaturationLimit=inf  LowerSaturationLimit=-inf  LinearizeAsGain=off  AntiWindupMode=none  Kb=1  TrackingMode=off  Kt=1  PParamMin=[]  PParamMax=[]  IParamMin=[]  IParamMax=[]  DParamMin=[]  DParamMax=[]  NParamMin=[]  NParamMax=[]  KbParamMin=[]  KbParamMax=[]  KtParamMin=[]  KtParamMax=[]  POutMin=[]  POutMax=[]  IOutMin=[]  IOutMax=[]  DOutMin=[]  DOutMax=[]  NOutMin=[]  NOutMax=[]  KbOutMin=[]  KbOutMax=[]  KtOutMin=[]  KtOutMax=[]  IntegratorOutMin=[]  IntegratorOutMax=[]  FilterOutMin=[]  FilterOutMax=[]  SumOutMin=[]  SumOutMax=[]  SumI1OutMin=[]  SumI1OutMax=[]  SumI2OutMin=[]  SumI2OutMax=[]  SumI3OutMin=[]  SumI3OutMax=[]  SumDOutMin=[]  SumDOutMax=[]  SaturationOutMin=[]  SaturationOutMax=[]  IntegratorContinuousStateAttributes=''  IntegratorStateMustResolveToSignalObject=off  IntegratorRTWStateStorageClass=Auto  FilterContinuousStateAttributes=''  FilterStateMustResolveToSignalObject=off  FilterRTWStateStorageClass=Auto  DifferentiatorICPrevScaledInput=0  DifferentiatorOutMin=[]  DifferentiatorOutMax=[]
  Mux16 : Mux  Inputs=2
  Mux4 : Mux  Inputs=2
  Product : Product
  Scope1 : Scope  NumInputPorts=3
  Scope2 : Scope  NumInputPorts=3
  Sum1 : Sum  Inputs=+++
  Sum2 : Sum  Inputs=|+-
  Sum3 : Sum  Inputs=|+-
  Sum4 : Sum  Inputs=+-|
  Vleg regulator : simulink/Continuous/PID Controller  Controller=PI  TimeDomain=Discrete-time  SampleTime=-1  IntegratorMethod=Forward Euler  FilterMethod=Forward Euler  Form=Parallel  UseFilter=on  ControllerParametersSource=external  P=8  I=0.5  D=0  N=100  InitialConditionSource=internal  InitialConditionForIntegrator=0  InitialConditionForFilter=0  ExternalReset=level  LimitOutput=on  UpperSaturationLimit=10  LowerSaturationLimit=-10  LinearizeAsGain=off  AntiWindupMode=back-calculation  Kb=Ki_Vleg/Kp_Vleg  TrackingMode=off  Kt=1  PParamMin=[]  PParamMax=[]  IParamMin=[]  IParamMax=[]  DParamMin=[]  DParamMax=[]  NParamMin=[]  NParamMax=[]  KbParamMin=[]  KbParamMax=[]  KtParamMin=[]  KtParamMax=[]  POutMin=[]  POutMax=[]  IOutMin=[]  IOutMax=[]  DOutMin=[]  DOutMax=[]  NOutMin=[]  NOutMax=[]  KbOutMin=[]  KbOutMax=[]  KtOutMin=[]  KtOutMax=[]  IntegratorOutMin=[]  IntegratorOutMax=[]  FilterOutMin=[]  FilterOutMax=[]  SumOutMin=[]  SumOutMax=[]  SumI1OutMin=[]  SumI1OutMax=[]  SumI2OutMin=[]  SumI2OutMax=[]  SumI3OutMin=[]  SumI3OutMax=[]  SumDOutMin=[]  SumDOutMax=[]  SaturationOutMin=[]  SaturationOutMax=[]  IntegratorContinuousStateAttributes=''  IntegratorStateMustResolveToSignalObject=off  IntegratorRTWStateStorageClass=Auto  FilterContinuousStateAttributes=''  FilterStateMustResolveToSignalObject=off  FilterRTWStateStorageClass=Auto  DifferentiatorICPrevScaledInput=0  DifferentiatorOutMin=[]  DifferentiatorOutMax=[]
  Edc : Outport
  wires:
  Vdc/1 -> Sum4/1, Divide/1, Product/1
  [PID_reset] -> Vleg regulator/4
  Ibus regulator/1 -> Scope1/3, Sum4/2
  I_bal/1 -> Sum1/3
  [Kp_Ibus_reg] -> Ibus regulator/2
  Pff/1 -> Divide/2
  Vleg regulator/1 -> Sum1/2, Scope2/3
  [Ki_Vleg_reg] -> Vleg regulator/3
  Decoupling5/1 -> Sum1/1
  Mux4/1 -> Scope1/1
  Sum3/1 -> Scope1/2, Ibus regulator/1
  Sum2/1 -> Vleg regulator/1, Scope2/2
  Product/1 -> Decoupling4/1
  Decoupling4/1 -> Mux16/1, Sum2/1
  Sum1/1 -> Sum3/1, Mux4/1  "Ibus_ref"
  Sum4/1 -> Edc/1  "Edc"
  [DC_boost_ratio] -> Product/2
  Vsm_avg/1 -> Mux16/2, Sum2/2
  Divide/1 -> Decoupling5/1
  Mux16/1 -> Scope2/1
  Ibus/1 -> Sum3/2, Mux4/2
  [Kp_Vleg_reg] -> Vleg regulator/2

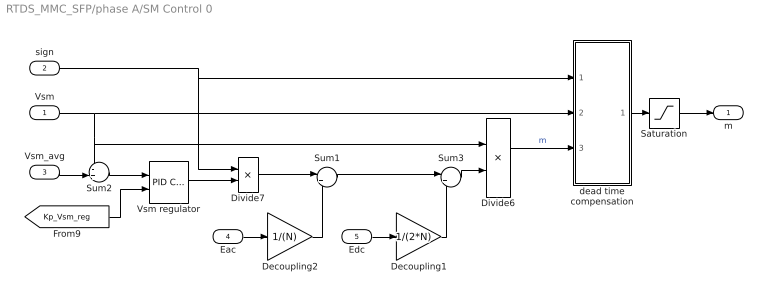
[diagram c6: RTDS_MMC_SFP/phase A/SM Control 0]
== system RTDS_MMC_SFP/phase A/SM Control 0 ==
  Vsm : Inport
  sign : Inport  Port=2
  Vsm_avg : Inport  Port=3
  Eac : Inport  Port=4
  Edc : Inport  Port=5
  Decoupling1 : Gain  Gain=1/(2*N)
  Decoupling2 : Gain  Gain=1/(N)
  Divide6 : Product  Inputs=/*
  Divide7 : Product  Inputs=**
  Saturation : Saturate  UpperLimit=0.95  LowerLimit=0.05
  Sum1 : Sum  Inputs=|++
  Sum2 : Sum  Inputs=-+|
  Sum3 : Sum  Inputs=|++
  Vsm regulator : simulink/Continuous/PID Controller  Controller=P  TimeDomain=Discrete-time  SampleTime=-1  IntegratorMethod=Forward Euler  FilterMethod=Forward Euler  Form=Parallel  UseFilter=on  ControllerParametersSource=external  P=8  I=0.5  D=0  N=100  InitialConditionSource=internal  InitialConditionForIntegrator=0  InitialConditionForFilter=0  ExternalReset=none  LimitOutput=off  UpperSaturationLimit=inf  LowerSaturationLimit=-inf  LinearizeAsGain=off  AntiWindupMode=none  Kb=1  TrackingMode=off  Kt=1  PParamMin=[]  PParamMax=[]  IParamMin=[]  IParamMax=[]  DParamMin=[]  DParamMax=[]  NParamMin=[]  NParamMax=[]  KbParamMin=[]  KbParamMax=[]  KtParamMin=[]  KtParamMax=[]  POutMin=[]  POutMax=[]  IOutMin=[]  IOutMax=[]  DOutMin=[]  DOutMax=[]  NOutMin=[]  NOutMax=[]  KbOutMin=[]  KbOutMax=[]  KtOutMin=[]  KtOutMax=[]  IntegratorOutMin=[]  IntegratorOutMax=[]  FilterOutMin=[]  FilterOutMax=[]  SumOutMin=[]  SumOutMax=[]  SumI1OutMin=[]  SumI1OutMax=[]  SumI2OutMin=[]  SumI2OutMax=[]  SumI3OutMin=[]  SumI3OutMax=[]  SumDOutMin=[]  SumDOutMax=[]  SaturationOutMin=[]  SaturationOutMax=[]  IntegratorContinuousStateAttributes=''  IntegratorStateMustResolveToSignalObject=off  IntegratorRTWStateStorageClass=Auto  FilterContinuousStateAttributes=''  FilterStateMustResolveToSignalObject=off  FilterRTWStateStorageClass=Auto  DifferentiatorICPrevScaledInput=0  DifferentiatorOutMin=[]  DifferentiatorOutMax=[]
  dead time compensation : Subsystem
  m : Outport
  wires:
  [Kp_Vsm_reg] -> Vsm regulator/2
  Sum2/1 -> Vsm regulator/1
  sign/1 -> dead time compensation/1(sign), Divide7/1
  Vsm regulator/1 -> Divide7/2
  Vsm/1 -> dead time compensation/2(Vdc), Divide6/1, Sum2/1
  Vsm_avg/1 -> Sum2/2
  Sum3/1 -> Divide6/2
  Saturation/1 -> m/1
  Divide6/1 -> dead time compensation/3(m)  "m"
  dead time compensation/1(m') -> Saturation/1
  Divide7/1 -> Sum1/1
  Sum1/1 -> Sum3/1
  Eac/1 -> Decoupling2/1
  Decoupling2/1 -> Sum1/2
  Edc/1 -> Decoupling1/1
  Decoupling1/1 -> Sum3/2

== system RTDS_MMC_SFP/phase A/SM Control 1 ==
  Vsm : Inport
  sign : Inport  Port=2
  Vsm_avg : Inport  Port=3
  Eac : Inport  Port=4
  Edc : Inport  Port=5
  Decoupling1 : Gain  Gain=1/(2*N)
  Decoupling2 : Gain  Gain=1/(N)
  Divide6 : Product  Inputs=/*
  Divide7 : Product  Inputs=**
  Saturation : Saturate  UpperLimit=0.95  LowerLimit=0.05
  Sum1 : Sum  Inputs=|++
  Sum2 : Sum  Inputs=-+|
  Sum3 : Sum  Inputs=|++
  Vsm regulator : simulink/Continuous/PID Controller  Controller=P  TimeDomain=Discrete-time  SampleTime=-1  IntegratorMethod=Forward Euler  FilterMethod=Forward Euler  Form=Parallel  UseFilter=on  ControllerParametersSource=external  P=8  I=0.5  D=0  N=100  InitialConditionSource=internal  InitialConditionForIntegrator=0  InitialConditionForFilter=0  ExternalReset=none  LimitOutput=off  UpperSaturationLimit=inf  LowerSaturationLimit=-inf  LinearizeAsGain=off  AntiWindupMode=none  Kb=1  TrackingMode=off  Kt=1  PParamMin=[]  PParamMax=[]  IParamMin=[]  IParamMax=[]  DParamMin=[]  DParamMax=[]  NParamMin=[]  NParamMax=[]  KbParamMin=[]  KbParamMax=[]  KtParamMin=[]  KtParamMax=[]  POutMin=[]  POutMax=[]  IOutMin=[]  IOutMax=[]  DOutMin=[]  DOutMax=[]  NOutMin=[]  NOutMax=[]  KbOutMin=[]  KbOutMax=[]  KtOutMin=[]  KtOutMax=[]  IntegratorOutMin=[]  IntegratorOutMax=[]  FilterOutMin=[]  FilterOutMax=[]  SumOutMin=[]  SumOutMax=[]  SumI1OutMin=[]  SumI1OutMax=[]  SumI2OutMin=[]  SumI2OutMax=[]  SumI3OutMin=[]  SumI3OutMax=[]  SumDOutMin=[]  SumDOutMax=[]  SaturationOutMin=[]  SaturationOutMax=[]  IntegratorContinuousStateAttributes=''  IntegratorStateMustResolveToSignalObject=off  IntegratorRTWStateStorageClass=Auto  FilterContinuousStateAttributes=''  FilterStateMustResolveToSignalObject=off  FilterRTWStateStorageClass=Auto  DifferentiatorICPrevScaledInput=0  DifferentiatorOutMin=[]  DifferentiatorOutMax=[]
  dead time compensation : Subsystem
  m : Outport
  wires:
  Decoupling1/1 -> Sum3/2
  Edc/1 -> Decoupling1/1
  Decoupling2/1 -> Sum1/2
  Eac/1 -> Decoupling2/1
  Sum1/1 -> Sum3/1
  Divide7/1 -> Sum1/1
  dead time compensation/1(m') -> Saturation/1
  Divide6/1 -> dead time compensation/3(m)  "m"
  Saturation/1 -> m/1
  Sum3/1 -> Divide6/2
  Vsm_avg/1 -> Sum2/2
  Vsm/1 -> Sum2/1, Divide6/1, dead time compensation/2(Vdc)
  Vsm regulator/1 -> Divide7/2
  sign/1 -> Divide7/1, dead time compensation/1(sign)
  Sum2/1 -> Vsm regulator/1
  [Kp_Vsm_reg] -> Vsm regulator/2

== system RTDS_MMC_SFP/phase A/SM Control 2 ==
  Vsm : Inport
  sign : Inport  Port=2
  Vsm_avg : Inport  Port=3
  Eac : Inport  Port=4
  Edc : Inport  Port=5
  Decoupling1 : Gain  Gain=1/(2*N)
  Decoupling2 : Gain  Gain=1/(N)
  Divide6 : Product  Inputs=/*
  Divide7 : Product  Inputs=**
  Saturation : Saturate  UpperLimit=0.95  LowerLimit=0.05
  Sum1 : Sum  Inputs=|++
  Sum2 : Sum  Inputs=-+|
  Sum3 : Sum  Inputs=|++
  Vsm regulator : simulink/Continuous/PID Controller  Controller=P  TimeDomain=Discrete-time  SampleTime=-1  IntegratorMethod=Forward Euler  FilterMethod=Forward Euler  Form=Parallel  UseFilter=on  ControllerParametersSource=external  P=8  I=0.5  D=0  N=100  InitialConditionSource=internal  InitialConditionForIntegrator=0  InitialConditionForFilter=0  ExternalReset=none  LimitOutput=off  UpperSaturationLimit=inf  LowerSaturationLimit=-inf  LinearizeAsGain=off  AntiWindupMode=none  Kb=1  TrackingMode=off  Kt=1  PParamMin=[]  PParamMax=[]  IParamMin=[]  IParamMax=[]  DParamMin=[]  DParamMax=[]  NParamMin=[]  NParamMax=[]  KbParamMin=[]  KbParamMax=[]  KtParamMin=[]  KtParamMax=[]  POutMin=[]  POutMax=[]  IOutMin=[]  IOutMax=[]  DOutMin=[]  DOutMax=[]  NOutMin=[]  NOutMax=[]  KbOutMin=[]  KbOutMax=[]  KtOutMin=[]  KtOutMax=[]  IntegratorOutMin=[]  IntegratorOutMax=[]  FilterOutMin=[]  FilterOutMax=[]  SumOutMin=[]  SumOutMax=[]  SumI1OutMin=[]  SumI1OutMax=[]  SumI2OutMin=[]  SumI2OutMax=[]  SumI3OutMin=[]  SumI3OutMax=[]  SumDOutMin=[]  SumDOutMax=[]  SaturationOutMin=[]  SaturationOutMax=[]  IntegratorContinuousStateAttributes=''  IntegratorStateMustResolveToSignalObject=off  IntegratorRTWStateStorageClass=Auto  FilterContinuousStateAttributes=''  FilterStateMustResolveToSignalObject=off  FilterRTWStateStorageClass=Auto  DifferentiatorICPrevScaledInput=0  DifferentiatorOutMin=[]  DifferentiatorOutMax=[]
  dead time compensation : Subsystem
  m : Outport
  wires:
  [Kp_Vsm_reg] -> Vsm regulator/2
  Sum2/1 -> Vsm regulator/1
  sign/1 -> dead time compensation/1(sign), Divide7/1
  Vsm regulator/1 -> Divide7/2
  Vsm/1 -> dead time compensation/2(Vdc), Divide6/1, Sum2/1
  Vsm_avg/1 -> Sum2/2
  Sum3/1 -> Divide6/2
  Saturation/1 -> m/1
  Divide6/1 -> dead time compensation/3(m)  "m"
  dead time compensation/1(m') -> Saturation/1
  Divide7/1 -> Sum1/1
  Sum1/1 -> Sum3/1
  Eac/1 -> Decoupling2/1
  Decoupling2/1 -> Sum1/2
  Edc/1 -> Decoupling1/1
  Decoupling1/1 -> Sum3/2
